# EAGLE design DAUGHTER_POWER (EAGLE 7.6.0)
DAUGHTER CARD POWER

## Sheet 1 of 3: HDK INTERFACE
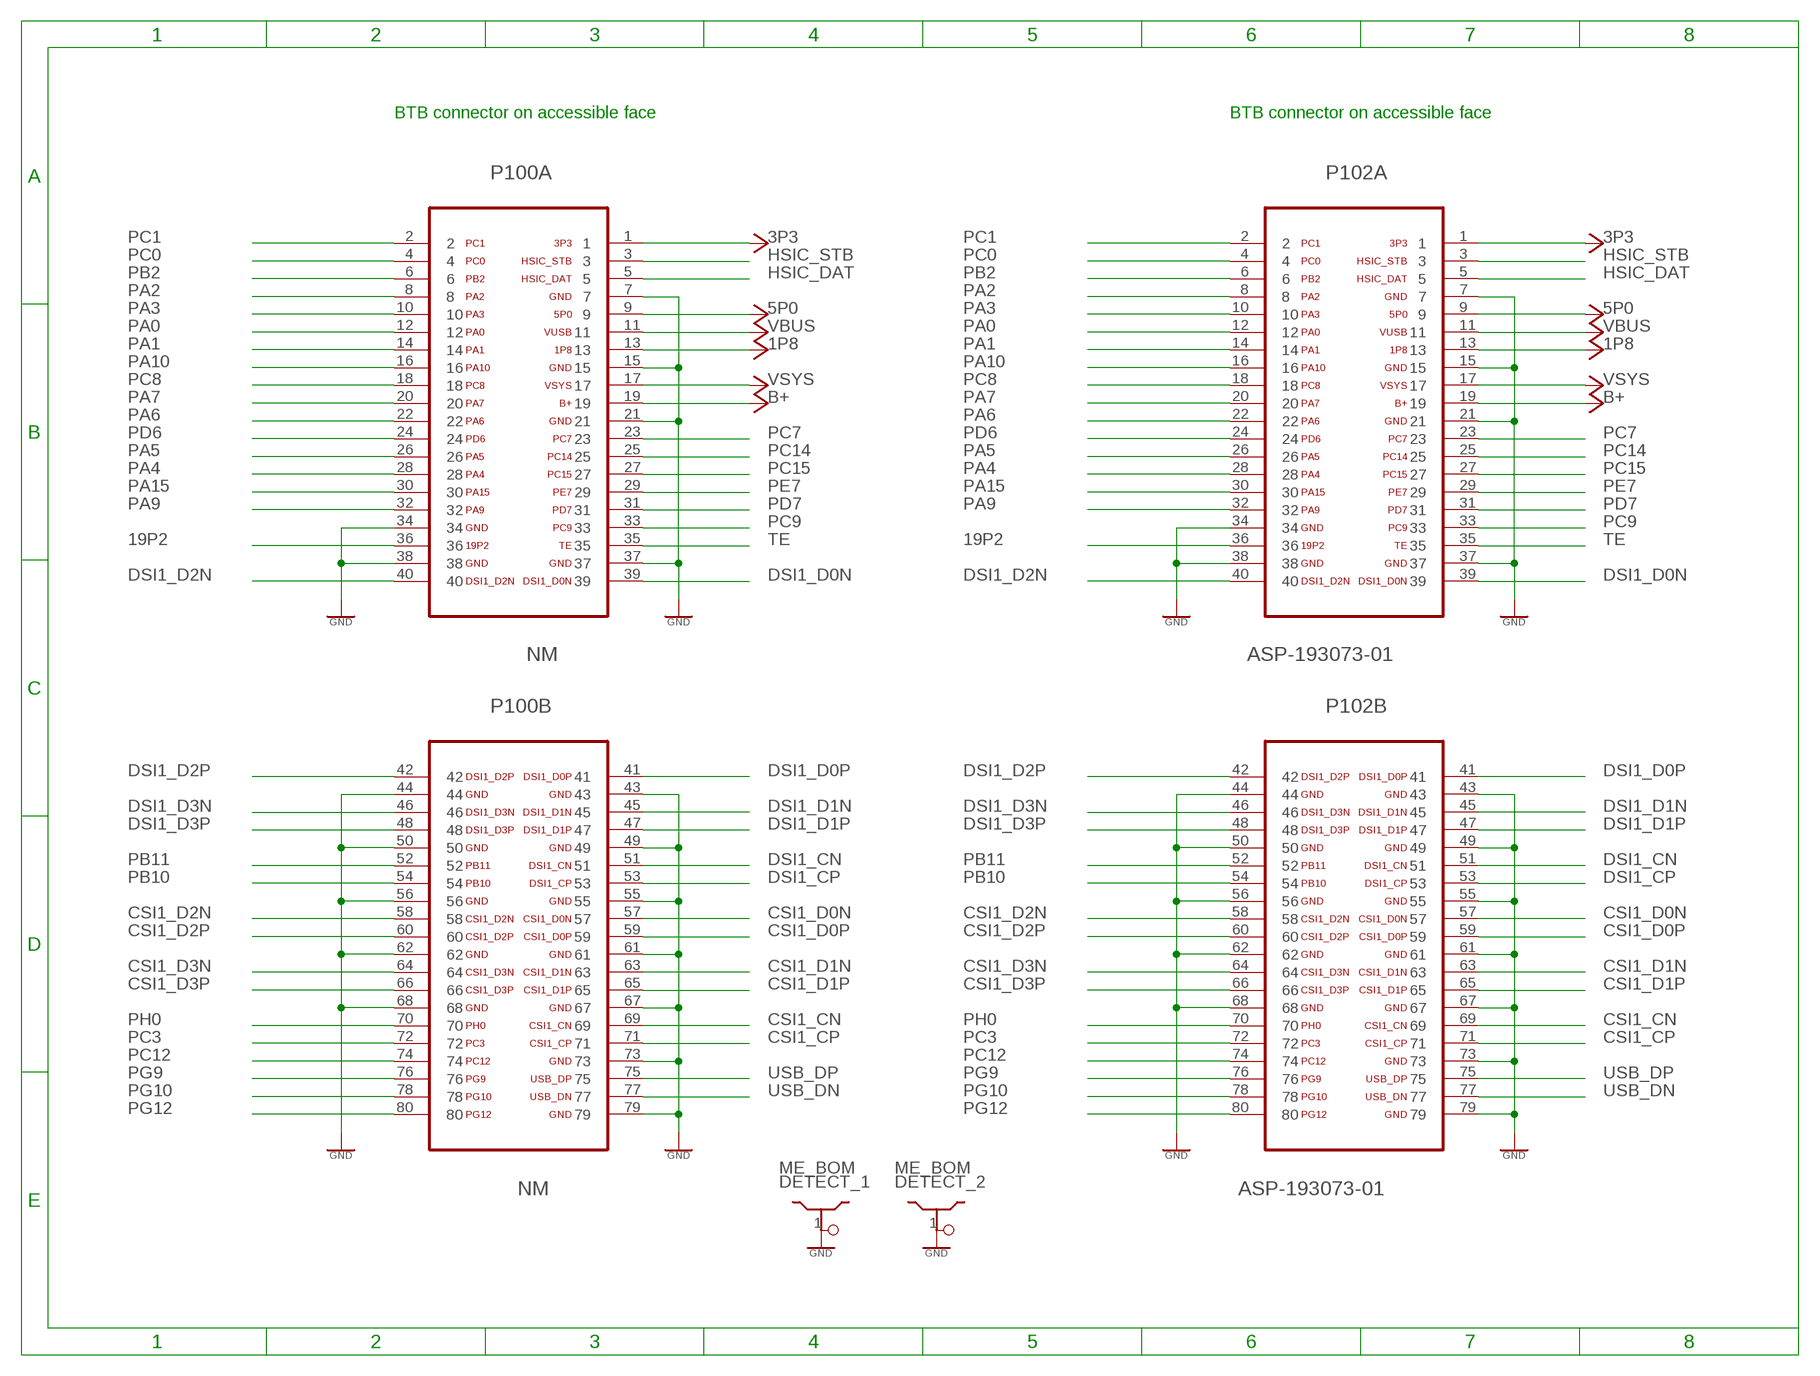
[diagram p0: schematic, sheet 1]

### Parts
DETECT_1  ME_BOM  SHIELDDETECT  [PLUG]
DETECT_2  ME_BOM  SHIELDDETECT  [PLUG]
P100  NM  CLM-140-02-L-D-KGOLD  [CLM-140-02-L-D-K_GOLD]
P102  ASP-193073-01  FTMH-140-02-L-DV-ES-P-TR  [FTMH-140-02-L-DV-ES-P-TR]

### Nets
1P8: P100.13 P102.13 ; also sheet 2,3
3P3: P100.1 P102.1 ; also sheet 2
5P0: P100.9 P102.9
19P2: P100.36 P102.36
B+: P100.19 P102.19
CSI1_CN: P100.69 P102.69
CSI1_CP: P100.71 P102.71
CSI1_D0N: P100.57 P102.57
CSI1_D0P: P100.59 P102.59
CSI1_D1N: P100.63 P102.63
CSI1_D1P: P100.65 P102.65
CSI1_D2N: P100.58 P102.58
CSI1_D2P: P100.60 P102.60
CSI1_D3N: P100.64 P102.64
CSI1_D3P: P100.66 P102.66
DSI1_CN: P100.51 P102.51
DSI1_CP: P100.53 P102.53
DSI1_D0N: P100.39 P102.39
DSI1_D0P: P100.41 P102.41
DSI1_D1N: P100.45 P102.45
DSI1_D1P: P100.47 P102.47
DSI1_D2N: P100.40 P102.40
DSI1_D2P: P100.42 P102.42
DSI1_D3N: P100.46 P102.46
DSI1_D3P: P100.48 P102.48
GND: DETECT_1.1 DETECT_2.1 P100.7 P100.15 P100.21 P100.34 P100.37 P100.38 P100.43 P100.44 P100.49 P100.50 P100.55 P100.56 P100.61 P100.62 P100.67 P100.68 P100.73 P100.79 P102.7 P102.15 P102.21 P102.34 P102.37 P102.38 P102.43 P102.44 P102.49 P102.50 P102.55 P102.56 P102.61 P102.62 P102.67 P102.68 P102.73 P102.79 ; also sheet 2,3
HSIC_DAT: P100.5 P102.5
HSIC_STB: P100.3 P102.3
PA0: P100.12 P102.12
PA1: P100.14 P102.14
PA2: P100.8 P102.8
PA3: P100.10 P102.10
PA4: P100.28 P102.28
PA5: P100.26 P102.26
PA6: P100.22 P102.22
PA7: P100.20 P102.20
PA9: P100.32 P102.32
PA10: P100.16 P102.16
PA15: P100.30 P102.30
PB2: P100.6 P102.6 ; also sheet 3
PB10: P100.54 P102.54 ; also sheet 2,3
PB11: P100.52 P102.52 ; also sheet 2,3
PC0: P100.4 P102.4
PC1: P100.2 P102.2
PC3: P100.72 P102.72
PC7: P100.23 P102.23 ; also sheet 3
PC8: P100.18 P102.18
PC9: P100.33 P102.33
PC12: P100.74 P102.74
PC14: P100.25 P102.25
PC15: P100.27 P102.27
PD6: P100.24 P102.24
PD7: P100.31 P102.31
PE7: P100.29 P102.29
PG9: P100.76 P102.76 ; also sheet 2
PG10: P100.78 P102.78 ; also sheet 3
PG12: P100.80 P102.80 ; also sheet 3
PH0: P100.70 P102.70
TE: P100.35 P102.35
USB_DN: P100.77 P102.77
USB_DP: P100.75 P102.75
VBUS: P100.11 P102.11 ; also sheet 3
VSYS: P100.17 P102.17 ; also sheet 3

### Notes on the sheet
- BTB connector on accessible face | BTB connector on accessible face

## Sheet 2 of 3: Identification
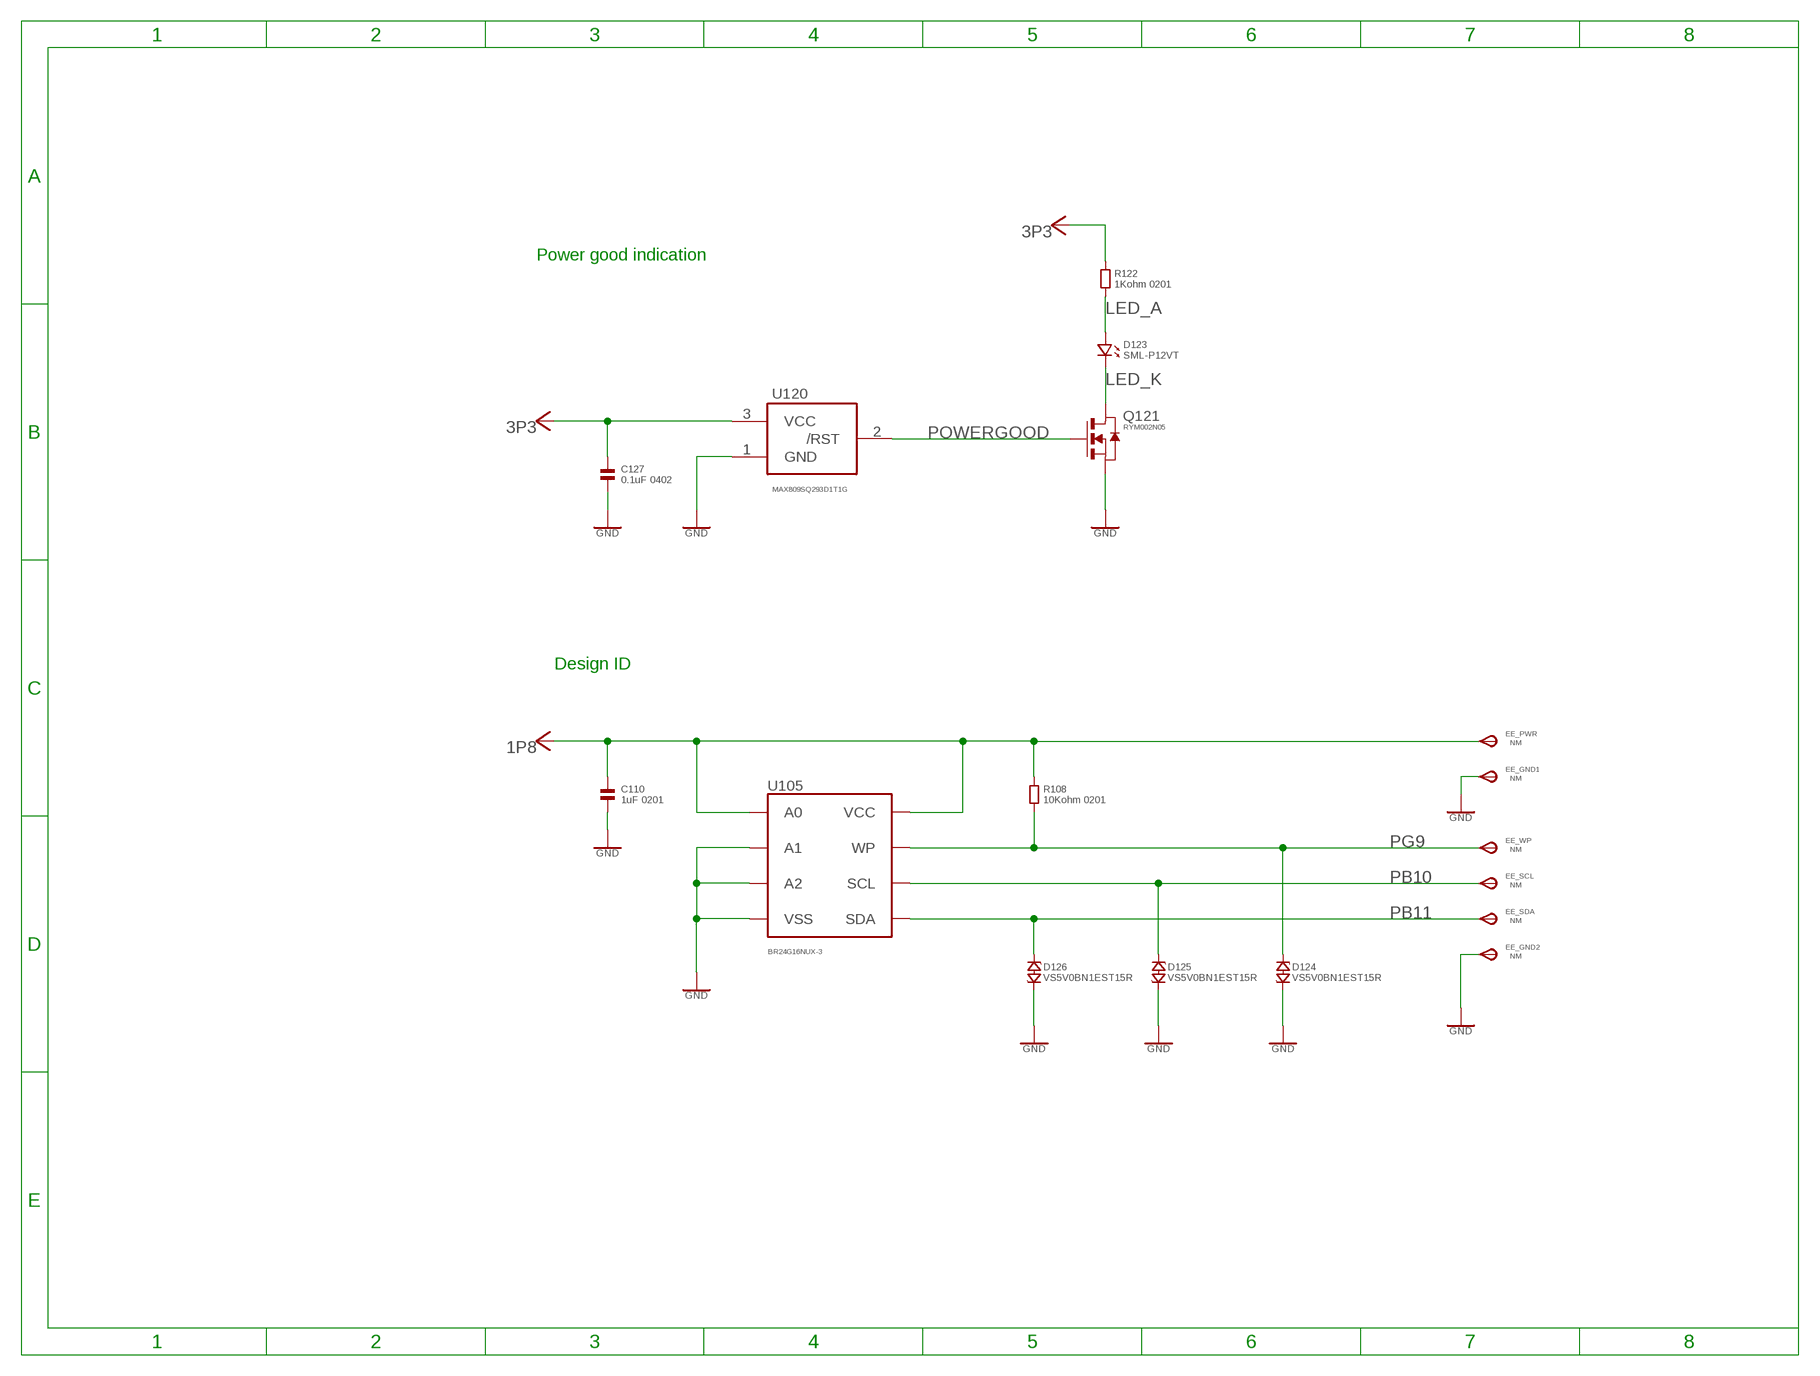
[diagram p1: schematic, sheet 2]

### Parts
C110  1uF 0201  CAPACITOR.0201  [0201]
C127  0.1uF 0402  CAPACITOR.0402  [0402]
D123  SML-P12VT  LED.0503  [0503.LED]
D124  VS5V0BN1EST15R  ESD_VARISTOR.0201  [CHIP_0201]
D125  VS5V0BN1EST15R  ESD_VARISTOR.0201  [CHIP_0201]
D126  VS5V0BN1EST15R  ESD_VARISTOR.0201  [CHIP_0201]
EE_GND1  NM  TPSTP11R  [TP11R]
EE_GND2  NM  TPSTP11R  [TP11R]
EE_PWR  NM  TPSTP11R  [TP11R]
EE_SCL  NM  TPSTP11R  [TP11R]
EE_SDA  NM  TPSTP11R  [TP11R]
EE_WP  NM  TPSTP11R  [TP11R]
Q121  RYM002N05  FET-NRYM002N05  [VMT3]
R108  10Kohm 0201  RESISTOR.0201  [0201]
R122  1Kohm 0201  RESISTOR.0201  [0201]
U105  BR24G16NUX-3  EEPROMDFN8  [DFN-8]
U120  MAX809SQ293D1T1G  MAX809  [SC70-3L]

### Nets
1P8: C110.1 EE_PWR.TP(PP) R108.1 U105.P$1(A0) U105.P$8(VCC) ; also sheet 1,3
3P3: C127.1 R122.1 U120.3(VCC) ; also sheet 1
GND: C110.2 C127.2 D124.P$2 D125.P$2 D126.P$2 EE_GND1.TP(PP) EE_GND2.TP(PP) Q121.2(S) U105.P$2(A1) U105.P$3(A2) U105.P$4(VSS) U105.P$9(VSS) U120.1(GND) ; also sheet 1,3
LED_A: D123.P$1 R122.2
LED_K: D123.P$2 Q121.3(D)
PB10: D125.P$1 EE_SCL.TP(PP) U105.P$6(SCL) ; also sheet 1,3
PB11: D126.P$1 EE_SDA.TP(PP) U105.P$5(SDA) ; also sheet 1,3
PG9: D124.P$1 EE_WP.TP(PP) R108.2 U105.P$7(WP) ; also sheet 1
POWERGOOD: Q121.1(G) U120.2(/RST)

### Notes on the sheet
- Power good indication
- Design ID

## Sheet 3 of 3: BATTERY
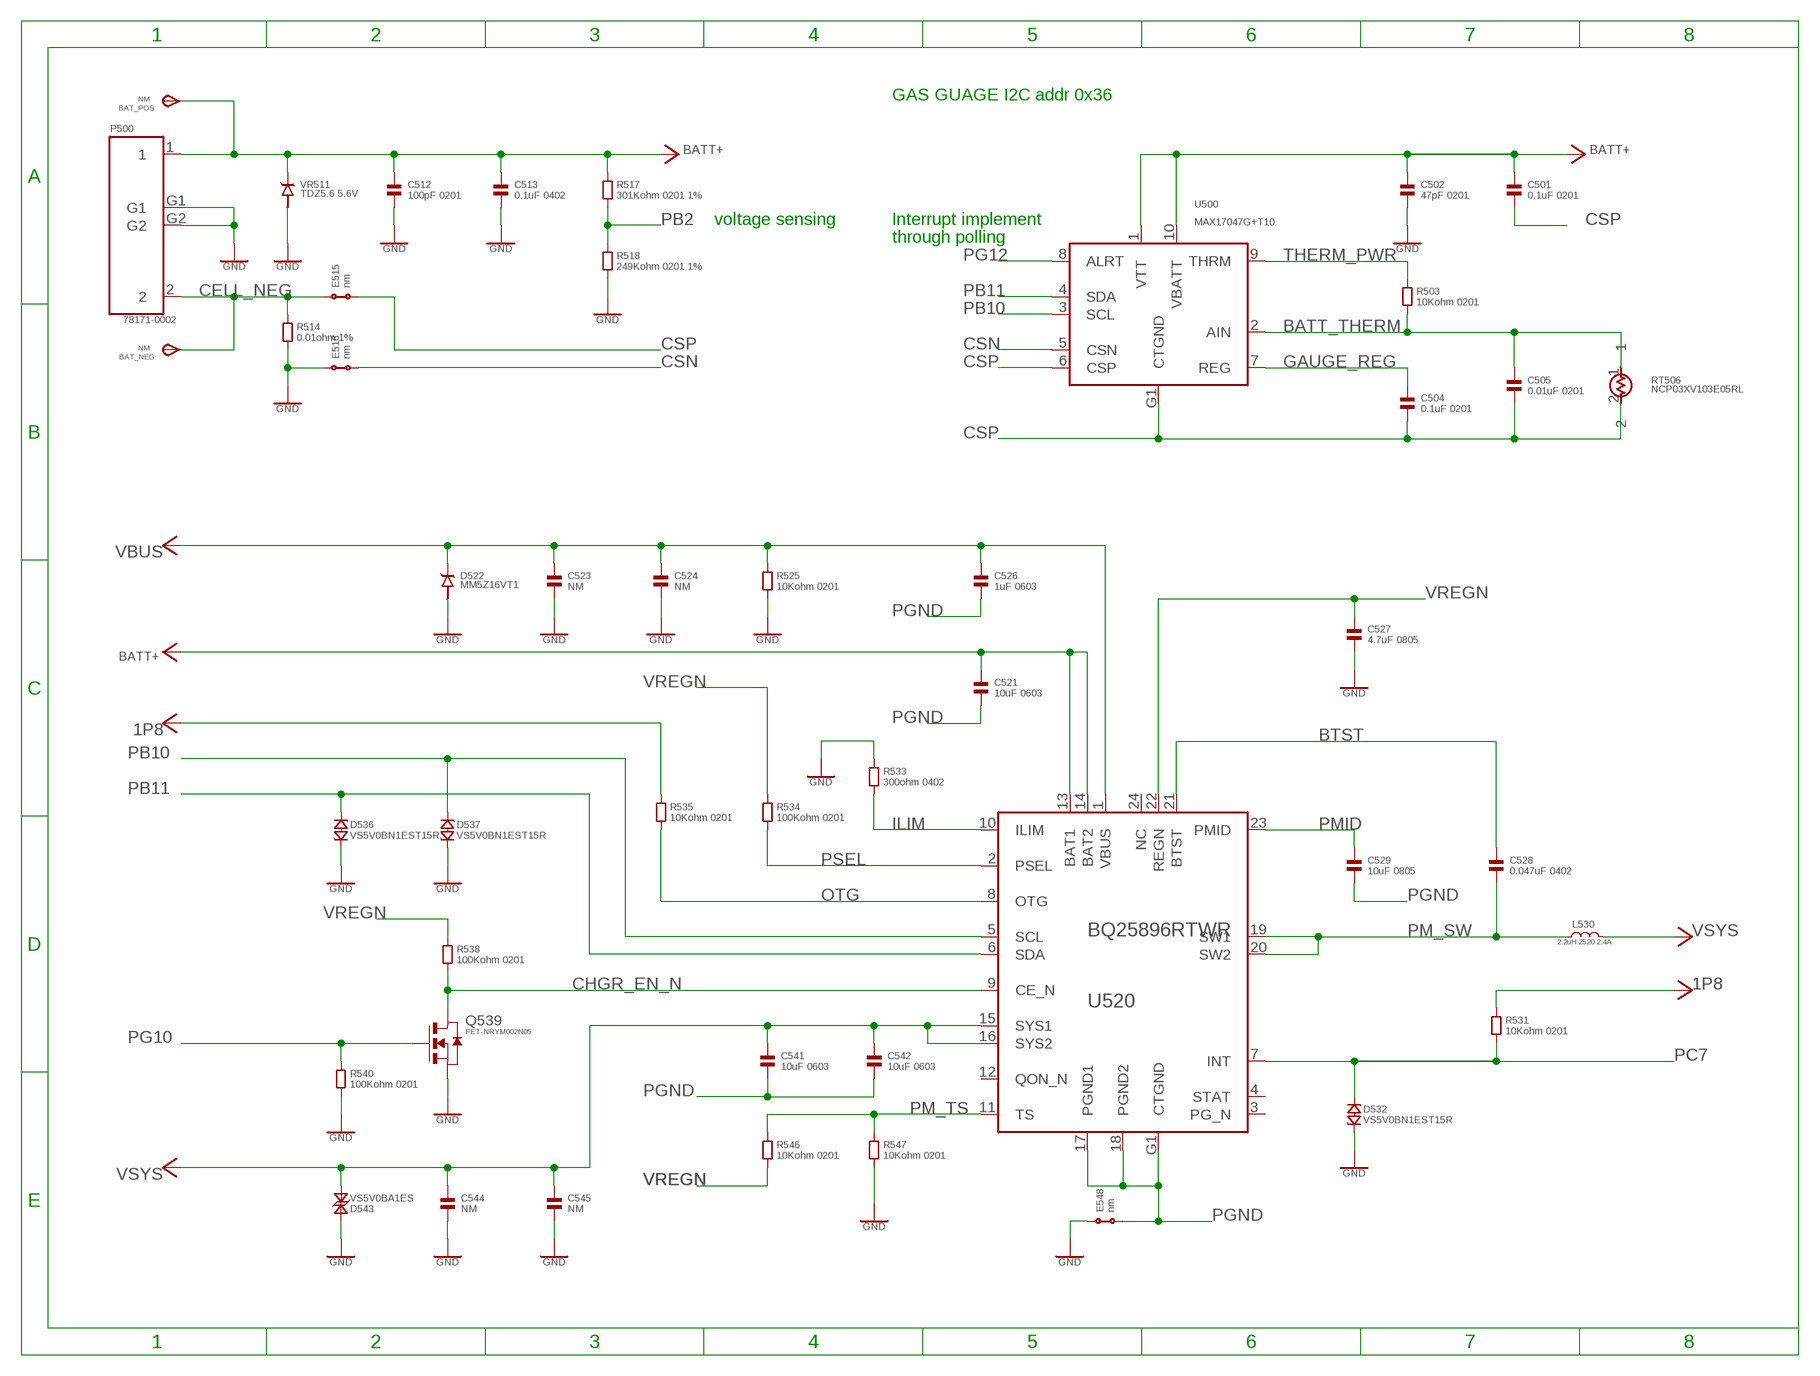
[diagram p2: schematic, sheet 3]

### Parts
BAT_NEG  NM  TPSTP11R  [TP11R]
BAT_POS  NM  TPSTP11R  [TP11R]
C501  0.1uF 0201  CAPACITOR.0201  [0201]
C502  47pF 0201  CAPACITOR.0201  [0201]
C504  0.1uF 0201  CAPACITOR.0201  [0201]
C505  0.01uF 0201  CAPACITOR.0201  [0201]
C512  100pF 0201  CAPACITOR.0201  [0201]
C513  0.1uF 0402  CAPACITOR.0402  [0402]
C521  10uF 0603  CAPACITOR.0603  [0603]
C523  NM  CAPACITOR.0201  [0201]
C524  NM  CAPACITOR.0201  [0201]
C526  1uF 0603  CAPACITOR.0603  [0603]
C527  4.7uF 0805  CAPACITOR.0805  [0805]
C528  0.047uF 0402  CAPACITOR.0402  [0402]
C529  10uF 0805  CAPACITOR.0805  [0805]
C541  10uF 0603  CAPACITOR.0603  [0603]
C542  10uF 0603  CAPACITOR.0603  [0603]
C544  NM  CAPACITOR.0201  [0201]
C545  NM  CAPACITOR.0201  [0201]
D522  MM5Z16VT1  DIODE.SOD523  [SOD523]
D532  VS5V0BN1EST15R  ESD_VARISTOR.0201  [CHIP_0201]
D536  VS5V0BN1EST15R  ESD_VARISTOR.0201  [CHIP_0201]
D537  VS5V0BN1EST15R  ESD_VARISTOR.0201  [CHIP_0201]
D543  VS5V0BA1ES  ESD_TVS.0201  [CHIP_0201]
E515  nm  SHORT_DOT  [SHORT_DOT]
E516  nm  SHORT_DOT  [SHORT_DOT]
E548  nm  SHORT_BAR  [1X4_SHORT]
L530  2.2uH 2520 2.4A  POWER-INDUCTOR  [2520]
P500  78171-0002  CONN_BATT  [CONN_4PIN]
Q539  FET-NRYM002N05  [VMT3]
R503  10Kohm 0201  RESISTOR.0201  [0201]
R514  0.01ohm 1%  RESISTOR.0805  [0805]
R517  301Kohm 0201 1%  RESISTOR.0201  [0201]
R518  249Kohm 0201 1%  RESISTOR.0201  [0201]
R525  10Kohm 0201  RESISTOR.0201  [0201]
R531  10Kohm 0201  RESISTOR.0201  [0201]
R533  300ohm 0402  RESISTOR.0402  [0402]
R534  100Kohm 0201  RESISTOR.0201  [0201]
R535  10Kohm 0201  RESISTOR.0201  [0201]
R538  100Kohm 0201  RESISTOR.0201  [0201]
R540  100Kohm 0201  RESISTOR.0201  [0201]
R546  10Kohm 0201  RESISTOR.0201  [0201]
R547  10Kohm 0201  RESISTOR.0201  [0201]
RT506  NCP03XV103E05RL  THERMISTOR  [0201]
U500  MAX17047G+T10  [DFN3X3_PS0_5P11]
U520  BQ25896RTWR  [QFN4X4PS0_5P25]
VR511  TDZ5.6 5.6V  DIODE  [DIO1_9X1_3]

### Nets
1P8: R531.1 R535.1 ; also sheet 1,2
BATT+: BAT_POS.TP(PP) C501.1 C502.1 C512.1 C513.1 C521.1 P500.1 R517.1 U500.1(VTT) U500.10(VBATT) U520.13(BAT1) U520.14(BAT2) VR511.1
BATT_THERM: C505.1 R503.2 RT506.1 U500.2(AIN)
BTST: C528.1 U520.21(BTST)
CELL_NEG: BAT_NEG.TP(PP) E515.1 P500.2 R514.1
CHGR_EN_N: Q539.3(D) R538.2 U520.9(CE_N)
CSN: E516.2 U500.5(CSN)
CSP: C501.2 C504.2 C505.2 E515.2 RT506.2 U500.6(CSP) U500.G1(CTGND)
GAUGE_REG: C504.1 U500.7(REG)
GND: C502.2 C512.2 C513.2 C523.2 C524.2 C527.2 C544.2 C545.2 D522.2 D532.P$2 D536.P$2 D537.P$2 D543.P$1 E516.1 E548.1 P500.G1 P500.G2 Q539.2(S) R514.2 R518.2 R525.2 R533.1 R540.2 R547.2 VR511.2 ; also sheet 1,2
ILIM: R533.2 U520.10(ILIM)
OTG: R535.2 U520.8(OTG)
PB2: R517.2 R518.1 ; also sheet 1
PB10: D537.P$1 U500.3(SCL) U520.5(SCL) ; also sheet 1,2
PB11: D536.P$1 U500.4(SDA) U520.6(SDA) ; also sheet 1,2
PC7: D532.P$1 R531.2 U520.7(INT) ; also sheet 1
PG10: Q539.1(G) R540.1 ; also sheet 1
PG12: U500.8(ALRT) ; also sheet 1
PGND: C521.2 C526.2 C529.2 C541.2 C542.2 E548.2 U520.17(PGND1) U520.18(PGND2) U520.G1(CTGND)
PM_SW: C528.2 L530.G1 U520.19(SW1) U520.20(SW2)
PM_TS: R546.1 R547.1 U520.11(TS)
PMID: C529.1 U520.23(PMID)
PSEL: R534.2 U520.2(PSEL)
THERM_PWR: R503.1 U500.9(THRM)
VBUS: C523.1 C524.1 C526.1 D522.1 R525.1 U520.1(VBUS) ; also sheet 1
VREGN: C527.1 R534.1 R538.1 R546.2 U520.22(REGN)
VSYS: C541.1 C542.1 C544.1 C545.1 D543.P$2 L530.G2 U520.15(SYS1) U520.16(SYS2) ; also sheet 1
Unconnected: U520.3(PG_N) U520.4(STAT) U520.12(QON_N) U520.24(NC)

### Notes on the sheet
- GAS GUAGE I2C addr 0x36
- voltage sensing | Interrupt implement
- through polling

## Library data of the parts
BAT_NEG BAT_POS EE_GND1 EE_GND2 EE_PWR EE_SCL EE_SDA EE_WP = MOTO_LIB:TPS: TEST Point, 1mm diameter, gold
C110 C127 C501 C502 C504 C505 C512 C513 C521 C523 C524 C526-C529 C541 C542 C544 C545 = MOTO_LIB:CAPACITOR: Ceramic Capacitor, Generic
D123 = MOTO_LIB:LED: LED GENERIC, single, 2 pin; MPN: SML-P12VT; SUPPLIER: ROHM
D124-D126 D532 D536 D537 = MOTO_LIB:ESD_VARISTOR: GENERIC varistor,single, 2 pin; MPN: VS5V0BN1EST15R; SUPPLIER: ROHM
D522 = MOTO_LIB:DIODE: DIODE GENERIC, single, 2 pin; MPN: MM5Z16VT1; SUPPLIER: ON_SEMI
D543 = MOTO_LIB:ESD_TVS: GENERIC TVS,single, 2 pin; MPN: UCLAMP1211Z; SUPPLIER: SEMTECH
DETECT_1 DETECT_2 = MOTO_LIB:SHIELD: Shield, Custom; MPN: refer to ME BOM; SUPPLIER: ref to ME BOM
E515 E516 = MOTO_LIB:SHORT_DOT: short dot, layout feature
E548 = MOTO_LIB:SHORT_BAR: SHORT BAR - layout feature
L530 = MOTO_LIB:POWER-INDUCTOR: Inductor, Power
P100 = MOTO_LIB:CLM-140-02-L-D-K: MICRO SOCKET, 1.0MM pitch, SMD, 2X40WAY, Female; MPN: CLM-140-02-L-D-K; SUPPLIER: SAMTEC
P102 = MOTO_LIB:FTMH-140-02-L-DV-ES-P-TR: MICRO SOCKET, 1.0MM, SMD, 2X40WAY, MALE; MPN: ASP-193073-01; SUPPLIER: SAMTEC
P500 = MOTO_LIB:CONN_BATT: BATTERY connector; MPN: 78171-0002; SUPPLIER: MOLEX
Q121 Q539 = MOTO_LIB:FET-N: Generic NMOS FET; MPN: RYM002N05; SUPPLIER: ROHM
R108 R122 R503 R514 R517 R518 R525 R531 R533-R535 R538 R540 R546 R547 = MOTO_LIB:RESISTOR: Resistor - Generic
RT506 = MOTO_LIB:THERMISTOR: Thmistor, NTC 10Khm 3%, 0201; MPN: NCP03XV103XV103E05RL/NTCG0603UH103HT; SUPPLIER: MURARA/TDK
U105 = MOTO_LIB:EEPROM: I2C EE PROM, 8 pin; MPN: BR24G16NUX-3; SUPPLIER: ROHM
U120 = MOTO_LIB:MAX809: 3-Pin Microprocessor Reset Circuit; MPN: MAX809SQ293D1T1; SUPPLIER: ON-SEMI
U500 = MOTO_LIB:MAX17047G+T10: Fuel Guage; MPN: MAX17047G+T10; SUPPLIER: MAXIM
U520 = MOTO_LIB:BQ25896RTWR: Charging IC, TI BQ2589x; MPN: BQ25896RTWR; SUPPLIER: TI
VR511 = MOTO_LIB:DIODE: DIODE GENERIC, single, 2 pin; MPN: TDZ5.6B; SUPPLIER: ROHM

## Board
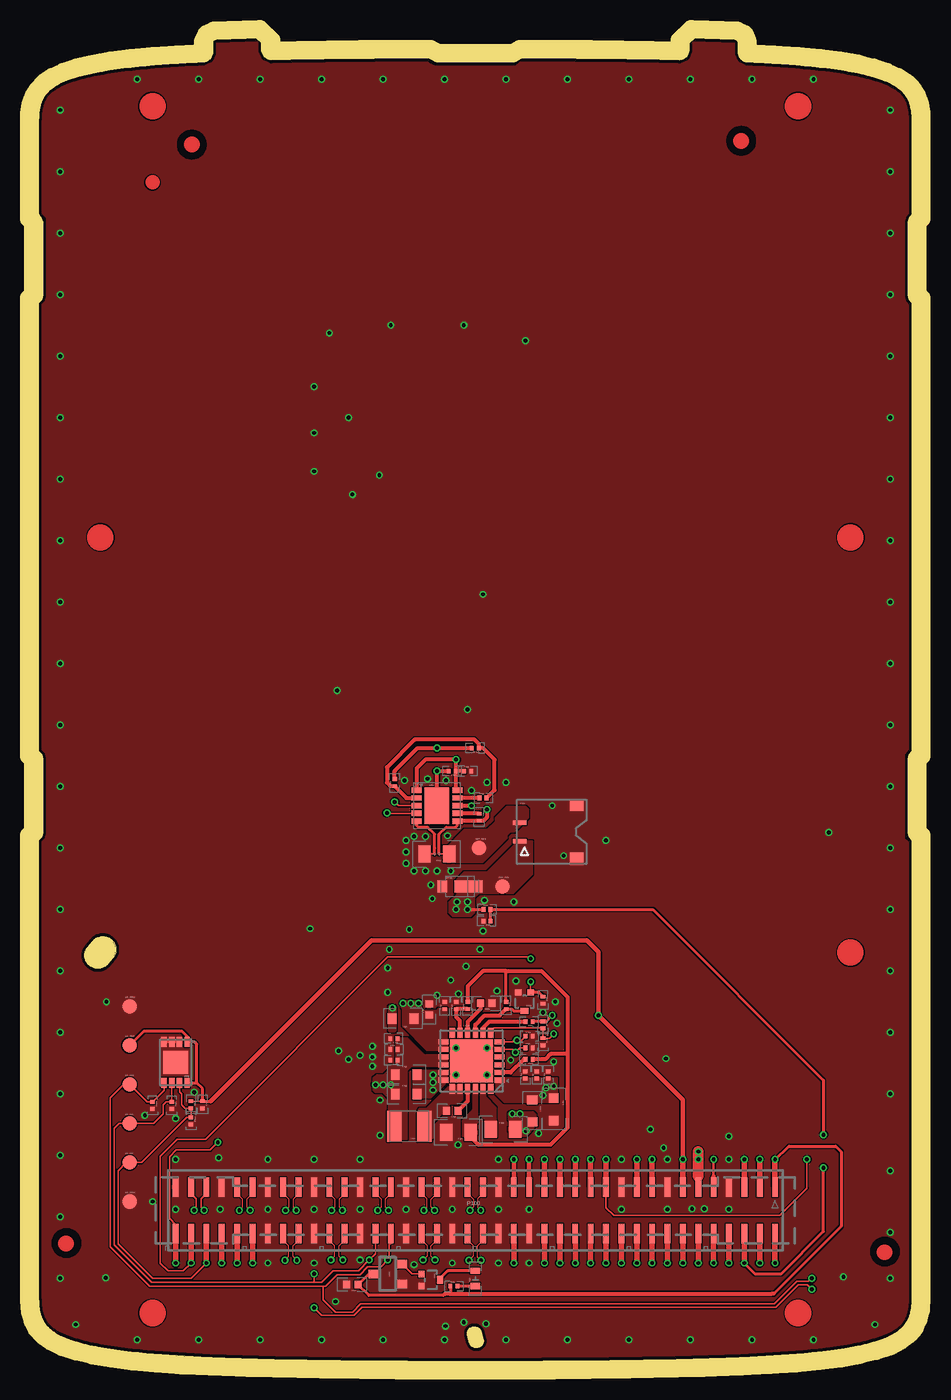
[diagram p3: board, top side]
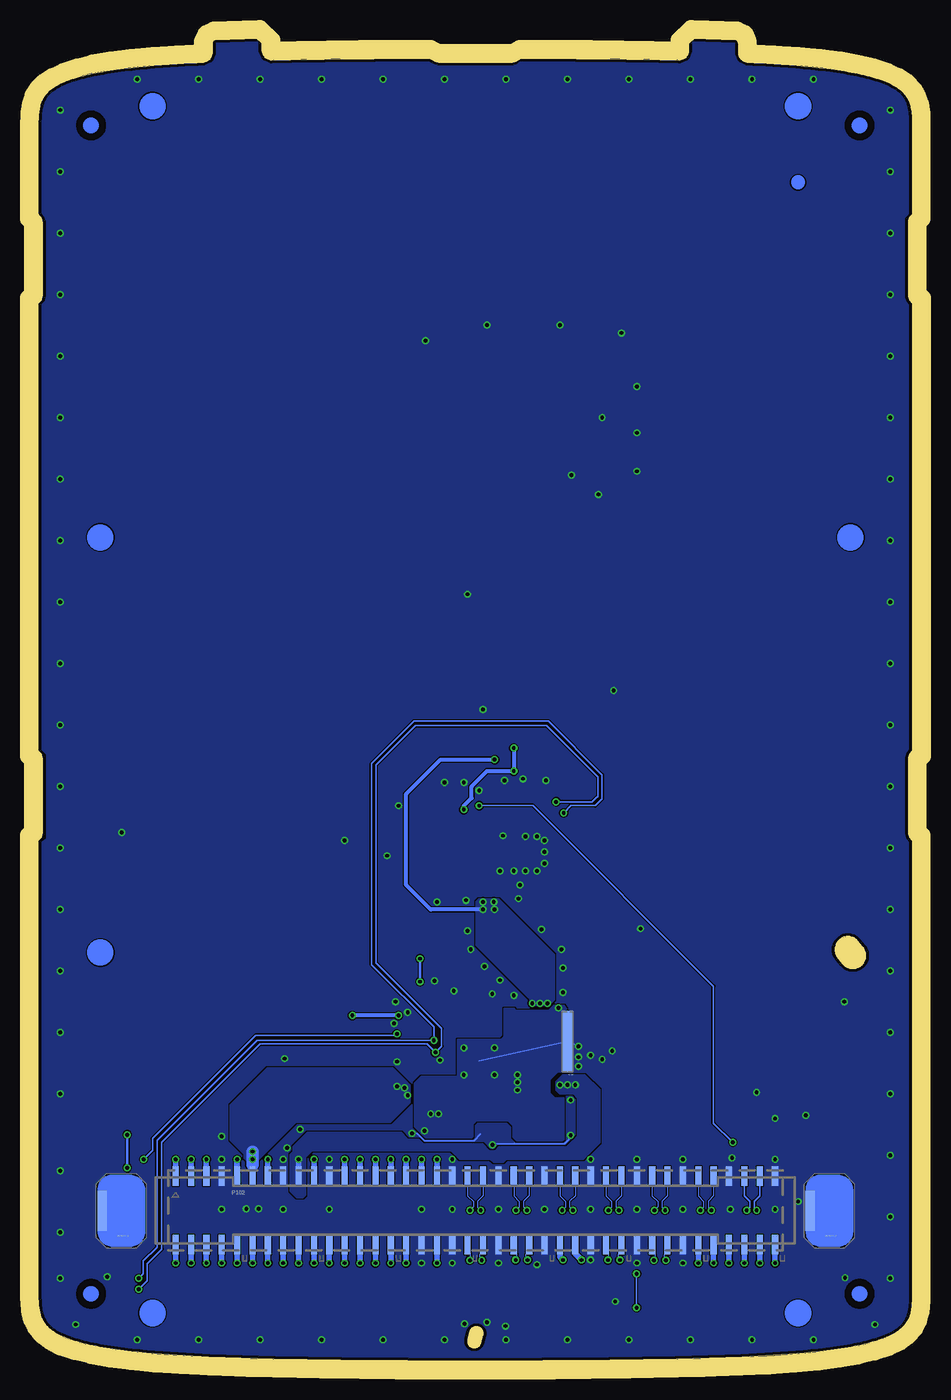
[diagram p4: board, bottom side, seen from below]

Size 56.85 x 86.03 mm. Coordinates in mm from the lower left corner, seen from the top.
Outline: 357 segments
Copper layers (1*16): Top 0.03mm / dielectric 0.787mm / Bottom 0.03mm
Design rules "constraint *": minimum track width 0.08mm, minimum drill 0.25mm, track to track 0.08mm, track to pad 0.08mm, pad to pad 0.08mm, via to via 0.08mm, smd to smd 0.08mm, copper to edge 0.2mm, drill to drill 0.2mm, minimum pad ring 0.1mm, minimum via ring 0.1mm, stop-mask expansion 0mil, vias tented up to drill 0.25mm, thermal gap 0mil
tRestrict: area 54.2,6.2 to 56,7.1; area 54.2,7.1 to 56,8; area 44.8,79.4 to 46.6,80.3; area 44.8,78.5 to 46.6,79.4; area 9.1,79.1 to 10.9,80; area 9.1,78.2 to 10.9,79.1; area 0.9,6.8 to 2.7,7.7; area 0.9,7.7 to 2.7,8.6
bRestrict: area 52.5,4.4 to 54.3,5.3; area 52.5,3.5 to 54.3,4.4; area 2.5,4.4 to 4.3,5.3; area 2.5,3.5 to 4.3,4.4; area 2.5,79.5 to 4.3,80.4; area 2.5,80.4 to 4.3,81.3; area 52.5,80.4 to 54.3,81.3; area 52.5,79.5 to 54.3,80.4
Milling: 125 lines

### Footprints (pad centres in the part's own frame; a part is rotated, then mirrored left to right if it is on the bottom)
TP11R = smd 0.95 x 0.95: TP 0,0
0201 = smd 0.25 x 0.3: 1 -0.23,0; 2 0.23,0
0402 = smd 0.45 x 0.5: 1 -0.37,0; 2 0.37,0
0603 = smd 0.58 x 0.68: 1 -0.71,0; 2 0.71,0
0805 = smd 0.8 x 1.1: 1 -0.8,0; 2 0.8,0
0503.LED = smd 0.4 x 0.6: P$1 -0.495,0; P$2 0.495,0
CHIP_0201 = smd 0.25 x 0.3: P$1 -0.23,0; P$2 0.23,0
SOD523 = smd 0.64 x 0.59: 1 -0.73,0; 2 0.73,0
PLUG = smd 0.6 x 2.6: 1 -1.25,0
SHORT_DOT = smd 0.05 x 0.05: 1 -0.01,0; 2 0.01,0
1X4_SHORT = smd 0.4 x 4: 1 -0.15,0; 2 0.15,0
2520 = smd 0.95 x 2: G1 -0.975,0; G2 0.975,0
CLM-140-02-L-D-K_GOLD = smd 0.38 x 1.27: 1 19.5,1.52; 2 19.5,-1.52; 3 18.5,1.52; 4 18.5,-1.52; 5 17.5,1.52; 6 17.5,-1.52; 7 16.5,1.52; 8 16.5,-1.52; 9 15.5,1.52; 10 15.5,-1.52; 11 14.5,1.52; 12 14.5,-1.52; 13 13.5,1.52; 14 13.5,-1.52; 15 12.5,1.52; 16 12.5,-1.52; 17 11.5,1.52; 18 11.5,-1.52; 19 10.5,1.52; 20 10.5,-1.52; 21 9.5,1.52; 22 9.5,-1.52; 23 8.5,1.52; 24 8.5,-1.52; 25 7.5,1.52; 26 7.5,-1.52; 27 6.5,1.52; 28 6.5,-1.52; 29 5.5,1.52; 30 5.5,-1.52; 31 4.5,1.52; 32 4.5,-1.52; 33 3.5,1.52; 34 3.5,-1.52; 35 2.5,1.52; 36 2.5,-1.52; 37 1.5,1.52; 38 1.5,-1.52; 39 0.5,1.52; 40 0.5,-1.52; 41 -0.5,1.52; 42 -0.5,-1.52; 43 -1.5,1.52; 44 -1.5,-1.52; 45 -2.5,1.52; 46 -2.5,-1.52; 47 -3.5,1.52; 48 -3.5,-1.52; 49 -4.5,1.52; 50 -4.5,-1.52; 51 -5.5,1.52; 52 -5.5,-1.52; 53 -6.5,1.52; 54 -6.5,-1.52; 55 -7.5,1.52; 56 -7.5,-1.52; 57 -8.5,1.52; 58 -8.5,-1.52; 59 -9.5,1.52; 60 -9.5,-1.52; 61 -10.5,1.52; 62 -10.5,-1.52; 63 -11.5,1.52; 64 -11.5,-1.52; 65 -12.5,1.52; 66 -12.5,-1.52; 67 -13.5,1.52; 68 -13.5,-1.52; 69 -14.5,1.52; 70 -14.5,-1.52; 71 -15.5,1.52; 72 -15.5,-1.52; 73 -16.5,1.52; 74 -16.5,-1.52; 75 -17.5,1.52; 76 -17.5,-1.52; 77 -18.5,1.52; 78 -18.5,-1.52; 79 -19.5,1.52; 80 -19.5,-1.52
FTMH-140-02-L-DV-ES-P-TR = smd 0.4 x 1.263: 1 -19.5,2.223; 2 -19.5,-2.223; 3 -18.5,2.223; 4 -18.5,-2.223; 5 -17.5,2.223; 6 -17.5,-2.223; 7 -16.5,2.223; 8 -16.5,-2.223; 9 -15.5,2.223; 10 -15.5,-2.223; 11 -14.5,2.223; 12 -14.5,-2.223; 13 -13.5,2.223; 14 -13.5,-2.223; 15 -12.5,2.223; 16 -12.5,-2.223; 17 -11.5,2.223; 18 -11.5,-2.223; 19 -10.5,2.223; 20 -10.5,-2.223; 21 -9.5,2.223; 22 -9.5,-2.223; 23 -8.5,2.223; 24 -8.5,-2.223; 25 -7.5,2.223; 26 -7.5,-2.223; 27 -6.5,2.223; 28 -6.5,-2.223; 29 -5.5,2.223; 30 -5.5,-2.223; 31 -4.5,2.223; 32 -4.5,-2.223; 33 -3.5,2.223; 34 -3.5,-2.223; 35 -2.5,2.223; 36 -2.5,-2.223; 37 -1.5,2.223; 38 -1.5,-2.223; 39 -0.5,2.223; 40 -0.5,-2.223; 41 0.5,2.223; 42 0.5,-2.223; 43 1.5,2.223; 44 1.5,-2.223; 45 2.5,2.223; 46 2.5,-2.223; 47 3.5,2.223; 48 3.5,-2.223; 49 4.5,2.223; 50 4.5,-2.223; 51 5.5,2.223; 52 5.5,-2.223; 53 6.5,2.223; 54 6.5,-2.223; 55 7.5,2.223; 56 7.5,-2.223; 57 8.5,2.223; 58 8.5,-2.223; 59 9.5,2.223; 60 9.5,-2.223; 61 10.5,2.223; 62 10.5,-2.223; 63 11.5,2.223; 64 11.5,-2.223; 65 12.5,2.223; 66 12.5,-2.223; 67 13.5,2.223; 68 13.5,-2.223; 69 14.5,2.223; 70 14.5,-2.223; 71 15.5,2.223; 72 15.5,-2.223; 73 16.5,2.223; 74 16.5,-2.223; 75 17.5,2.223; 76 17.5,-2.223; 77 18.5,2.223; 78 18.5,-2.223; 79 19.5,2.223; 80 19.5,-2.223
CONN_4PIN = smd 0.88 x 0.3: 1 -2.075,-0.6; 2 -2.075,0.6 | smd 0.9 x 0.8: G1 1.645,-1.75; G2 1.645,1.75
VMT3 = smd 0.42 x 0.4: 1 -0.4,-0.6; 2 0.4,-0.6 | smd 0.52 x 0.4: 3 0,0.6
DFN-8 = smd 0.35 x 0.65: P$1 -0.75,-1.325; P$2 -0.25,-1.325; P$3 0.25,-1.325; P$4 0.75,-1.325; P$5 0.75,1.325; P$6 0.25,1.325; P$7 -0.25,1.325; P$8 -0.75,1.325 | smd 1.6 x 1.5: P$9 0,0
SC70-3L = smd 0.55 x 0.63: 1 -0.65,-0.94; 3 0,0.94 | smd 0.555 x 0.63: 2 0.65,-0.94
DFN3X3_PS0_5P11 = smd 0.65 x 0.35: 1 -1.325,1; 2 -1.325,0.5; 3 -1.325,0; 4 -1.325,-0.5; 5 -1.325,-1; 6 1.325,-1; 7 1.325,-0.5; 8 1.325,0; 9 1.325,0.5; 10 1.325,1 | smd 1.6 x 2.4: G1 0,0
QFN4X4PS0_5P25 = smd 0.65 x 0.33: 1 1.825,-1.25; 2 1.825,-0.75; 3 1.825,-0.25; 4 1.825,0.25; 5 1.825,0.75; 6 1.825,1.25; 13 -1.825,1.25; 14 -1.825,0.75; 15 -1.825,0.25; 16 -1.825,-0.25; 17 -1.825,-0.75; 18 -1.825,-1.25 | smd 0.33 x 0.65: 7 1.25,1.825; 8 0.75,1.825; 9 0.25,1.825; 10 -0.25,1.825; 11 -0.75,1.825; 12 -1.25,1.825; 19 -1.25,-1.825; 20 -0.75,-1.825; 21 -0.25,-1.825; 22 0.25,-1.825; 23 0.75,-1.825; 24 1.25,-1.825 | smd 2.8 x 2.8: G1 0,0
DIO1_9X1_3 = smd 1.8 x 0.8: 1 0.55,0 | smd 0.6 x 0.8: 2 -1.15,0

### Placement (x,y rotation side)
BAT_NEG  28.67,33.37 0 top
BAT_POS  30.17,30.87 0 top
C110  10.67,16.67 270 top
C127  20.42,4.97 180 top
C501  26.92,38.37 180 top
C502  27.92,38.37 0 top
C504  28.67,35.37 270 top
C505  23.17,37.62 90 top
C512  26.42,23.12 90 top
C513  25.42,22.87 90 top
C521  23.72,22.27 180 top
C523  32.42,18.62 90 top
C524  31.67,18.62 90 top
C526  32.12,16.27 270 top
C527  27.32,14.87 180 top
C528  26.92,16.27 180 top
C529  30.22,15.07 0 top
C541  23.92,18.62 0 top
C542  23.92,17.37 0 top
C544  23.12,19.57 180 top
C545  23.12,20.97 180 top
D123  28.42,5.37 90 top
D124  9.92,15.62 270 top
D125  8.67,16.62 270 top
D126  7.42,16.62 270 top
D522  33.52,16.37 270 top
D532  32.82,20.77 270 top
D536  31.92,21.12 0 top
D537  31.92,20.37 0 top
D543  23.12,20.27 0 top
DETECT_1  51.45,9.77 0 bottom
DETECT_2  5.39,9.77 0 bottom
E515  26.07,32.97 0 top
E516  25.77,32.97 0 top
E548  22.42,20.77 180 bottom
EE_GND1  5.92,10.37 0 top
EE_GND2  5.92,23.07 0 top
EE_PWR  5.92,20.53 0 top
EE_SCL  5.92,15.45 0 top
EE_SDA  5.92,17.99 0 top
EE_WP  5.92,12.91 0 top
L530  24.12,15.27 180 top
P100  28.42,9.8 0 top
P102  28.42,9.8 0 bottom
P500  33.37,34.42 0 top
Q121  25.52,5.27 270 top
Q539  31.62,23.37 180 top
R108  9.92,16.67 270 top
R122  27.02,4.87 0 top
R503  28.92,36.62 0 top
R514  25.92,32.97 180 top
R517  29.17,29.37 0 top
R518  29.17,28.62 180 top
R525  33.17,18.62 90 top
R531  32.82,21.87 270 top
R533  29.12,23.27 180 top
R534  31.92,19.62 180 top
R535  31.92,22.07 180 top
R538  30.42,23.12 270 top
R540  32.82,23.47 270 top
R546  27.92,23.12 90 top
R547  27.17,23.12 90 top
RT506  28.42,39.87 180 top
U105  8.92,19.42 180 top
U120  22.72,5.67 90 top
U500  25.92,36.12 0 top
U520  28.17,19.52 0 top
VR511  27.42,30.87 0 top

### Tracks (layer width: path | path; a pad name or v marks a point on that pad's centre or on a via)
1P8  (via drill 0.25)
  Top 0.1: R108.1 C110.1
  Top 0.2: EE_PWR.TP 6.86,21.47 9.32,21.47 9.67,21.12 U105.P$1 10.15,20.75 10.3,20.6 10.3,18.1 | U105.P$8 10.3,18.1 | 10.3,18.1 10.67,17.72 C110.1 11.2,16.9 | R535.1 32.18,22.1 R531.1 33.05,22.1 v33.42,22.47
  Top 0.3: 11.2,16.9 21.67,27.37 35.67,27.37 36.42,26.62 v36.42,22.47 41.92,16.97 v41.92,13.12
  Top 0.35: P100.13 v41.92,13.12
  Bottom 0.25: v33.42,22.47 v36.42,22.47
  Bottom 0.35: P102.13 v41.92,13.12
3P3  (via drill 0.25)
  Top 0.2: U120.3 21.49,5.67 C127.1 21.49,4.27 26.32,4.27 26.42,4.37 | R122.1 26.79,4.37 | 47.92,13.07 48.82,13.97 51.87,13.97 52.22,13.62 52.22,8.77 47.83,4.38
  Top 0.25: 26.42,4.37 26.79,4.37 47.67,4.37 47.83,4.38
  Top 0.35: P100.1 v47.92,13.12 47.92,13.07
  Bottom 0.35: P102.1 v47.92,13.12
5P0  (via drill 0.25)
  Top 0.15: v43.92,13.12 P102.9
  Top 0.25: P100.9 P102.9
  Bottom 0.4: P102.9 v43.92,13.12
19P2  (via drill 0.25)
  Top 0.35: P100.36 v30.92,6.37
  Bottom 0.35: v30.92,6.37 P102.36
B+  (via drill 0.25)
  Top 0.35: P100.19 v38.92,13.12
  Bottom 0.35: v38.92,13.12 P102.19
BATT+  (via drill 0.25)
  Top 0.1: v27.17,39.12 27.15,39.1
  Top 0.2: v27.92,29.37 R517.1
  Top 0.25: U500.1 24.6,38.55 25.17,39.12 v27.17,39.12 | C501.1 27.15,39.1 | C501.1 27.15,37.22 U500.10 | C502.1 C501.1
  Bottom 0.25: v27.92,29.37 31.32,29.37 32.92,30.97 32.92,36.87 30.67,39.12 v27.17,39.12
  other vias: 27.92,29.87 27.22,29.87 27.17,29.37 23.72,23.27 24.22,23.27 24.72,23.27
  pour Bottom: 23.27,23.52 23.67,23.12 24.82,23.12 24.87,23.17 24.87,23.62 24.92,23.62 28.37,27.07 28.37,29.87 28.17,30.07 26.92,30.07 23.27,26.42
  pour Top: 32.12,33.82 30.97,33.82 30.97,33.57 29.22,31.82 27.72,31.82 27.22,31.32 27.22,30.32 26.72,29.82 26.72,29.17 26.97,28.92 28.12,28.92 28.37,29.17 28.37,30.17 28.62,30.42 30.87,30.42 32.12,31.67
  pour Top: 23.67,23.42 24.77,23.42 24.87,23.32 24.87,22.92 24.97,22.82 25.92,22.82 26.02,22.92 26.57,22.92 26.57,20.22 25.27,20.22 23.67,21.82 23.67,22.92 23.62,22.97 23.62,23.37
BATT_THERM
  Top 0.25: R503.2 29.67,37.14 29.67,39.12 28.92,39.87 RT506.1 28.65,40.14 28.37,40.42 24.47,40.42 22.67,38.62 22.67,37.62 22.9,37.39 C505.1 23.94,36.62 U500.2
BTST
  Top 0.25: U520.21 27.92,16.9 C528.1
CELL_NEG
  Top 0.1: E515.1 R514.1 E515.1
  pour Top: 27.72,34.57 29.22,34.57 29.72,35.07 29.72,35.32 30.47,36.07 31.67,36.07 31.87,35.87 31.87,35.37 30.92,34.42 30.67,34.42 30.47,34.22 30.47,34.02 28.87,32.42 26.47,32.42 26.47,33.32
CHGR_EN_N
  Top 0.2: R538.2 30.8,22.89 30.92,22.77 Q539.3
  Top 0.25: U520.9 28.42,21.87 29.02,22.47 30,22.47 R538.2
CSI1_CN  (via drill 0.25)
  Top 0.08: P100.69 13.92,10.9 13.57,10.55 13.57,10 v13.77,9.8
  Bottom 0.08: P102.69 13.92,10.75 13.57,10.4 13.57,10 v13.77,9.8
CSI1_CP  (via drill 0.25)
  Top 0.08: P100.71 12.92,10.9 13.29,10.53 13.29,10.02 v13.07,9.8
  Bottom 0.08: P102.71 12.92,10.75 13.27,10.4 13.27,10 v13.07,9.8
CSI1_D0N  (via drill 0.25)
  Top 0.08: P100.57 19.92,10.9 19.55,10.53 19.55,10.02 v19.77,9.8
  Bottom 0.08: P102.57 19.92,10.75 19.57,10.4 19.57,10 v19.77,9.8
CSI1_D0P  (via drill 0.25)
  Top 0.08: P100.59 18.92,10.9 19.27,10.55 19.27,10 v19.07,9.8
  Bottom 0.08: P102.59 18.92,10.75 19.29,10.38 19.29,10.02 v19.07,9.8
CSI1_D1N  (via drill 0.25)
  Top 0.08: P100.63 16.92,10.9 16.55,10.53 16.55,10.02 v16.77,9.8
  Bottom 0.08: P102.63 16.92,10.75 16.55,10.38 16.55,10.02 v16.77,9.8
CSI1_D1P  (via drill 0.25)
  Top 0.08: 15.92,10.9 16.27,10.55 16.27,10 v16.07,9.8
  Top 0.1: P100.65 15.92,10.9
  Bottom 0.08: P102.65 15.92,10.75 16.27,10.4 16.27,10 v16.07,9.8
CSI1_D2N  (via drill 0.25)
  Top 0.08: P100.58 19.92,7.85 19.57,7.5 19.57,6.8 v19.8,6.58
  Bottom 0.08: P102.58 19.92,7.17 19.72,6.97 19.72,6.65 v19.8,6.58
CSI1_D2P  (via drill 0.25)
  Top 0.08: P100.60 18.92,7.85 19.27,7.5 19.27,6.82 v19.03,6.58
  Bottom 0.08: P102.60 18.92,7.15 19.12,6.95 19.12,6.67 v19.03,6.58
CSI1_D3N  (via drill 0.25)
  Top 0.08: P100.64 16.92,7.85 16.57,7.5 16.57,6.8 v16.81,6.57
  Bottom 0.08: P102.64 16.92,7.12 16.72,6.92 16.72,6.65 v16.81,6.57
CSI1_D3P  (via drill 0.25)
  Top 0.08: P100.66 15.92,7.85 16.27,7.5 16.27,6.8 v16.03,6.57
  Bottom 0.08: P102.66 15.92,7.12 16.12,6.92 16.12,6.65 v16.03,6.57
CSN
  Top 0.1: E516.2 25.77,33.37
  Top 0.2: E516.2 25.77,33.37 25.77,34.27 25.32,34.72 24.72,34.72 24.6,34.85 U500.5
CSP  (via drill 0.25)
  Top 0.1: 27.27,35.14 U500.6 | E515.2
  Top 0.2: E515.2 26.07,34.27 26.52,34.72 27.12,34.72 27.25,34.85 U500.6
  Top 0.25: 27.27,35.14 C504.2 28.94,35.14 29.17,35.37 v29.17,35.87 | C501.2 v25.92,38.37 U500.G1 | RT506.2 v25.92,39.87 24.67,39.87 23.17,38.37 C505.2
  Bottom 0.25: v29.17,35.87 29.17,36.12 28.67,36.62 28.67,37.37 27.67,38.37 v25.92,38.37 v25.92,39.87
DSI1_CN  (via drill 0.25)
  Top 0.08: 22.92,10.9 22.55,10.53 22.55,10.02 v22.77,9.8
  Top 0.1: P100.51 22.92,10.9
  Bottom 0.08: P102.51 22.92,10.75 22.57,10.4 22.57,10 v22.77,9.8
DSI1_CP  (via drill 0.25)
  Top 0.08: P100.53 21.92,10.9 22.27,10.55 22.27,10 v22.07,9.8
  Bottom 0.08: P102.53 21.92,10.75 22.29,10.39 22.29,10.02 v22.07,9.8
DSI1_D0N  (via drill 0.25)
  Top 0.08: P100.39 28.92,10.9 28.57,10.55 28.57,10 v28.77,9.8
  Bottom 0.08: P102.39 28.92,10.75 28.55,10.38 28.55,10.02 v28.77,9.8
DSI1_D0P  (via drill 0.25)
  Top 0.08: P100.41 27.92,10.9 28.29,10.53 28.29,10.02 v28.07,9.8
  Bottom 0.08: P102.41 27.92,10.75 28.27,10.4 28.27,10 v28.07,9.8
DSI1_D1N  (via drill 0.25)
  Top 0.08: P100.45 25.92,10.9 25.55,10.53 25.55,10.02 v25.77,9.8
  Bottom 0.08: P102.45 25.92,10.75 25.57,10.4 25.57,10 v25.77,9.8
DSI1_D1P  (via drill 0.25)
  Top 0.08: P100.47 24.92,10.9 25.27,10.55 25.27,10 v25.07,9.8
  Bottom 0.08: P102.47 24.92,10.75 25.29,10.38 25.29,10.02 v25.07,9.8
DSI1_D2N  (via drill 0.25)
  Top 0.08: P100.40 28.92,7.85 28.57,7.5 28.57,6.76 v28.78,6.56
  Bottom 0.08: P102.40 28.92,7.17 28.72,6.97 28.72,6.61 v28.78,6.56
DSI1_D2P  (via drill 0.25)
  Top 0.08: P100.42 27.92,7.85 28.29,7.48 28.29,6.84 v28.01,6.56
  Bottom 0.08: P102.42 27.92,7.15 28.12,6.95 28.12,6.67 v28.01,6.56
DSI1_D3N  (via drill 0.25)
  Top 0.08: P100.46 25.92,7.87 25.56,7.5 25.55,6.82 v25.8,6.58
  Bottom 0.08: P102.46 25.92,7.17 25.72,6.97 25.72,6.65 v25.8,6.58
DSI1_D3P  (via drill 0.25)
  Top 0.08: P100.48 24.92,7.87 25.27,7.52 25.27,6.82 v25.03,6.58
  Bottom 0.08: P102.48 24.92,7.15 25.12,6.95 25.12,6.67 v25.03,6.58
GAUGE_REG
  Top 0.1: U500.7 27.42,35.6
  Top 0.25: C504.1 27.42,35.6 27.27,35.6
GND  (via drill 0.25)
  Top 0.1: E516.1 25.72,32.97 | 25.72,32.97 25.17,32.97 | 25.17,32.97 R514.2 | 25.72,32.97 E516.1 25.17,32.97
  Top 0.2: U105.P$4 U105.P$3 U105.P$2
  Bottom 0.1: v32.54,14.81 32.21,14.81 31.72,14.32 28.52,14.32 28.07,14.77 | v27.3,14.07 27.25,14.12 25.87,14.12 | 25.92,14.17 25.87,14.12 | 25.87,14.12 22.62,14.12 22.32,14.42 | E548.1 v21.72,20.47
  other vias: 14.42,1.37 10.42,1.37 6.42,1.37 22.42,1.37 18.42,1.37 26.42,1.37 30.42,1.37 34.42,1.37 38.42,1.37 42.42,1.37 46.42,1.37 50.42,1.37 54.42,2.37 55.42,8.37 55.42,5.37 55.42,12.37 55.42,17.37 55.42,21.37 55.42,25.37 55.42,29.37 55.42,33.37 55.42,37.37 55.42,41.37 55.42,45.37 55.42,49.37 55.42,53.37 55.42,57.37 55.42,61.37 55.42,65.37 55.42,69.37 55.42,73.37 55.42,77.37 55.42,81.37 50.42,83.37 46.42,83.37 42.42,83.37 38.42,83.37 34.42,83.37 30.42,83.37 26.42,83.37 22.42,83.37 18.42,83.37 14.42,83.37 10.42,83.37 6.42,83.37 1.42,81.37 1.42,77.37 1.42,73.37 1.42,69.37 1.42,65.37 1.42,61.37 1.42,57.37 1.42,53.37 1.42,49.37 1.42,45.37 1.42,41.37 1.42,37.37 1.42,33.37 1.42,29.37 1.42,25.37 4.42,23.37 1.42,21.37 1.42,17.37 1.42,13.37 1.42,9.37 1.42,5.37 2.42,2.37 8.92,13.12 11.72,13.22 14.92,13.12 17.92,13.12 20.92,13.12 29.92,13.12 29.92,9.87 31.92,9.87 26.92,9.87 23.92,9.87 20.92,9.87 17.92,9.87 14.92,9.87 11.82,9.87 8.92,9.87 7.42,10.37 8.92,15.77 10.12,17.47 14.92,6.37 17.92,6.37 20.92,6.57 24.42,6.27 26.92,6.37 29.92,6.37 31.92,6.37 44.92,9.87 42.52,9.9 43.32,9.9 40.92,9.87 37.92,9.87 37.92,13.12 40.92,13.12 44.92,13.12 6.92,15.97 29.12,2.42 27.67,2.52 26.47,2.27 52.37,5.47 4.37,5.42 31.67,66.37 27.67,67.37 22.92,67.37 18.92,66.87 17.92,63.37 17.92,60.37 20.17,61.37 17.92,57.87 20.42,56.37 22.17,57.62 28.92,49.87 27.92,42.37 19.42,43.62 29.17,37.62 30.42,37.62 36.92,33.87 26.82,31.87 28.17,37.12 33.42,36.12 34.17,32.87 25.17,34.12 24.42,34.12 23.92,33.87 23.92,33.12 23.92,32.37 24.42,31.87 25.17,31.87 25.92,31.87 30.92,29.87 23.82,37.77 25.32,37.87 26.52,37.77 26.62,34.17 25.52,30.97 25.62,30.07 24.12,28.07 22.82,26.77 22.72,25.57 29.02,29.97 28.92,27.97 28.72,26.77 27.82,25.67 29.82,24.07 31.07,24.72 27.32,23.87 26.82,24.77 25.92,23.77 22.72,23.97 20.92,19.87 20.17,19.62 19.52,20.17 30.72,19.57 33.52,19.47 33.62,23.37 32.82,22.67 33.72,21.97 22.22,16.97 22.22,14.67 39.82,15.07 40.67,13.87 40.82,19.67 44.92,14.62 51.42,34.37 19.32,3.87 17.67,28.12 21.72,19.77 21.72,19.17
  pour Top (rank 2): 25.82,84.22 31.07,84.22 31.57,84.67 36.72,84.67 41.82,84.57 42.12,84.67 42.32,84.97 42.42,85.17 42.42,85.57 42.72,85.97 45.32,85.87 45.42,85.67 45.42,84.97 45.62,84.57 45.82,84.47 46.12,84.37 47.12,84.37 50.02,84.17 51.72,83.97 53.32,83.67 54.82,83.27 55.72,82.87 56.22,82.47 56.52,82.07 56.72,81.47 56.82,80.77 56.82,74.97 56.42,74.47 56.32,74.07 56.32,69.27 56.42,68.87 56.82,68.47 56.82,39.97 56.32,39.47 56.32,33.97 56.82,33.57 56.82,4.87 56.72,3.47 56.52,2.67 56.12,2.17 55.52,1.77 54.22,1.27 52.92,0.97 51.62,0.77 48.72,0.47 44.72,0.27 43.62,0.27 43.32,0.37 38.32,0.27 38.02,0.17 36.62,0.07 20.12,0.07 18.72,0.17 18.52,0.27 13.52,0.37 13.22,0.27 10.82,0.37 7.02,0.57 3.92,0.97 2.32,1.37 1.32,1.77 0.72,2.17 0.42,2.47 0.22,2.97 0.12,3.47 0.02,4.47 0.02,33.57 0.42,33.97 0.52,34.27 0.52,39.27 0.32,39.67 0.12,39.97 0.02,40.07 0.02,68.47 0.32,68.77 0.52,69.17 0.52,74.37 0.02,74.87 0.02,80.27 0.12,81.27 0.42,82.27 0.72,82.57 1.72,83.17 3.02,83.57 4.52,83.87 7.02,84.17 9.92,84.37 10.82,84.37 11.22,84.57 11.42,84.87 11.42,85.67 11.52,85.87 14.12,85.97 14.42,85.67 14.42,85.07 14.62,84.77 14.92,84.57 15.52,84.57 19.92,84.67 25.17,84.67 25.37,84.42
  pour Bottom (rank 2): 25.82,84.27 31.02,84.27 31.42,84.47 31.62,84.67 36.72,84.67 41.82,84.57 42.12,84.67 42.32,84.97 42.42,85.17 42.42,85.57 42.72,85.97 45.32,85.87 45.42,85.67 45.42,84.97 45.62,84.57 45.82,84.47 46.12,84.37 47.12,84.37 50.02,84.17 51.72,83.97 53.32,83.67 54.82,83.27 55.72,82.87 56.22,82.47 56.52,82.07 56.72,81.47 56.82,80.77 56.82,74.97 56.42,74.47 56.32,74.07 56.32,69.27 56.42,68.87 56.82,68.47 56.82,39.97 56.32,39.47 56.32,33.97 56.82,33.57 56.82,4.87 56.72,3.47 56.52,2.67 56.12,2.17 55.52,1.77 54.22,1.27 52.92,0.97 51.62,0.77 48.72,0.47 44.72,0.27 43.62,0.27 43.32,0.37 38.32,0.27 38.02,0.17 36.62,0.07 20.12,0.07 18.72,0.17 18.52,0.27 13.52,0.37 13.22,0.27 10.82,0.37 7.02,0.57 3.92,0.97 2.32,1.37 1.32,1.77 0.72,2.17 0.42,2.47 0.22,2.97 0.12,3.47 0.02,4.47 0.02,33.57 0.42,33.97 0.52,34.27 0.52,39.27 0.32,39.67 0.12,39.97 0.02,40.07 0.02,68.47 0.32,68.77 0.52,69.17 0.52,74.37 0.02,74.87 0.02,80.27 0.12,81.27 0.42,82.27 0.72,82.57 1.72,83.17 3.02,83.57 4.52,83.87 7.02,84.17 9.92,84.37 10.82,84.37 11.22,84.57 11.42,84.87 11.42,85.67 11.52,85.87 14.12,85.97 14.42,85.67 14.42,85.07 14.62,84.77 14.92,84.57 15.52,84.57 19.92,84.67 25.32,84.67 25.62,84.37
HSIC_DAT  (via drill 0.25)
  Top 0.35: P100.5 v45.92,13.12
  Bottom 0.35: v45.92,13.12 P102.5
HSIC_STB  (via drill 0.25)
  Top 0.35: P100.3 v46.92,13.12
  Bottom 0.35: v46.92,13.12 P102.3
ILIM
  Top 0.1: R533.2
  Top 0.25: U520.10 27.92,22.07 28.76,22.91 R533.2
LED_A
  Top 0.1: R122.2
  Top 0.2: D123.P$1 R122.2
LED_K
  Top 0.2: D123.P$2 26.62,5.87 26.22,5.47 26.22,5.37 Q121.3
OTG
  Top 0.25: U520.8 28.92,21.67 29.32,22.07 R535.2
PA0  (via drill 0.25)
  Top 0.35: P100.12 v42.92,6.37
  Bottom 0.35: v42.92,6.37 P102.12
PA1  (via drill 0.25)
  Top 0.35: P100.14 v41.92,6.37
  Bottom 0.35: v41.92,6.37 P102.14
PA2  (via drill 0.25)
  Top 0.35: P100.8 v44.92,6.37
  Bottom 0.35: v44.92,6.37 P102.8
PA3  (via drill 0.25)
  Top 0.35: P100.10 v43.92,6.37
  Bottom 0.35: v43.92,6.37 P102.10
PA4  (via drill 0.25)
  Top 0.35: P100.28 v34.92,6.37
  Bottom 0.35: v34.92,6.37 P102.28
PA5  (via drill 0.25)
  Top 0.35: P100.26 v35.92,6.37
  Bottom 0.35: v35.92,6.37 P102.26
PA6  (via drill 0.25)
  Top 0.35: P100.22 v37.92,6.37
  Bottom 0.35: v37.92,6.37 P102.22
PA7  (via drill 0.25)
  Top 0.35: P100.20 v38.92,6.37
  Bottom 0.35: v38.92,6.37 P102.20
PA9  (via drill 0.25)
  Top 0.35: P100.32 v32.92,6.37
  Bottom 0.35: v32.92,6.37 P102.32
PA10  (via drill 0.25)
  Top 0.35: P100.16 v40.92,6.37
  Bottom 0.35: v40.92,6.37 P102.16
PA15  (via drill 0.25)
  Top 0.35: P100.30 v33.92,6.37
  Bottom 0.35: v33.92,6.37 P102.30
PB2  (via drill 0.25)
  Top 0.2: v45.92,6.37 46.62,5.67 48.32,5.67 51.07,8.42 v51.07,12.57 | v51.07,14.72 51.07,18.27 39.97,29.37 R517.2 R518.1
  Top 0.35: P100.6 v45.92,6.37
  Bottom 0.15: v51.07,14.72 v51.07,12.57
  Bottom 0.35: v45.92,6.37 P102.6
PB10  (via drill 0.25)
  Top 0.1: P100.54 21.92,6.97 v21.52,6.57 20.82,5.87 19.17,5.87 18.42,5.12 17.92,5.12 | 17.92,5.12 7.37,5.12 4.92,7.57 4.92,15.12 5.25,15.45 EE_SCL.TP 7.5,15.45 8.12,16.07 8.12,16.67 8.3,16.85 D125.P$1 U105.P$6 | v17.93,5.67 17.93,5.15 17.92,5.12 | v50.32,4.67 50.02,4.97 49.43,4.97 47.96,3.51 21.06,3.51 20.52,2.97 18.43,2.97 v17.93,3.47 | v23.17,36.37 23.42,36.12 U500.3 | U520.5 30.82,20.27 v31.02,20.07 31.32,20.37 D537.P$1
  Bottom 0.1: v23.17,36.37 20.82,36.37 20.51,36.69 20.46,36.69 20.46,38.01 23.79,41.34 32.31,41.34 34.89,38.76 34.89,25.89 30.62,21.62 30.62,20.47 v31.02,20.07 31.57,20.62 42.42,20.62 48.82,14.22 48.82,7.28 49.79,6.32 49.79,5.21 v50.32,4.67 | v17.93,5.67 v17.93,3.47
  Bottom 0.35: P102.54 21.92,6.97 v21.52,6.57
PB11  (via drill 0.25)
  Top 0.1: P100.52 22.92,7.67 22.82,7.57 22.82,6.67 v22.72,6.57 22.27,6.12 21.42,6.12 20.92,5.62 19.42,5.62 18.67,4.87 18.52,4.87 | 18.52,4.87 7.22,4.87 4.67,7.42 4.67,17.12 5.54,17.99 EE_SDA.TP 7.06,16.85 D126.P$1 8.17,17.6 U105.P$5 | v50.32,5.37 50.07,5.17 49.32,5.17 47.86,3.71 20.96,3.71 20.42,3.17 19.32,3.17 18.52,3.97 18.52,4.87 | U500.4 22.7,35.62 v22.67,35.65 | U520.6 30.84,20.77 30.93,20.86 v31.12,20.86 31.43,20.86 D536.P$1
  Bottom 0.1: v22.67,35.65 22.2,36.12 20.62,36.12 20.17,36.57 20.17,38.12 23.67,41.62 32.42,41.62 35.17,38.87 35.17,25.77 31.12,21.72 v31.12,20.86 42.61,20.86 49.12,14.35 49.12,7.41 50.02,6.51 50.02,5.67 v50.32,5.37
  Bottom 0.35: P102.52 22.92,6.77 v22.72,6.57
PC0  (via drill 0.25)
  Top 0.35: P100.4 v46.92,6.37
  Bottom 0.35: P102.4 v46.92,6.37
PC1  (via drill 0.25)
  Top 0.35: P100.2 v47.92,6.37
  Bottom 0.35: P102.2 v47.92,6.37
PC3  (via drill 0.25)
  Top 0.1: 12.92,8.87 P100.72 12.92,8.12
  Top 0.35: 12.92,8.12 v12.92,6.37
  Bottom 0.35: P102.72 v12.92,6.37
PC7  (via drill 0.25)
  Top 0.1: U520.7 29.42,21.47 29.62,21.67 32.42,21.67 | 32.42,21.67 32.79,21.67 | v33.52,21.27 33.25,21 D532.P$1 R531.2 32.42,21.67 | P100.23 36.92,9.97 37.42,9.47 48.22,9.47 50,11.25 v50,13.12
  Top 0.35: v36.92,13.12 P100.23
  Bottom 0.1: v33.52,21.27 33.62,21.17 42.72,21.17 49.42,14.47 49.42,13.7 v50,13.12
  Bottom 0.35: P102.23 v36.92,13.12
PC8  (via drill 0.25)
  Top 0.35: P100.18 v39.92,6.37
  Bottom 0.35: v39.92,6.37 P102.18
PC9  (via drill 0.25)
  Top 0.3: P100.33 v31.92,13.12
  Bottom 0.35: v31.92,13.12 P102.33
PC12  (via drill 0.25)
  Top 0.35: 11.92,8.37 P100.74 v11.92,6.37
  Bottom 0.35: P102.74 v11.92,6.37
PC14  (via drill 0.25)
  Top 0.35: P100.25 v35.92,13.12
  Bottom 0.35: v35.92,13.12 P102.25
PC15  (via drill 0.25)
  Top 0.35: P100.27 v34.92,13.12
  Bottom 0.35: v34.92,13.12 P102.27
PD6  (via drill 0.25)
  Top 0.35: P100.24 v36.92,6.37
  Bottom 0.35: v36.92,6.37 P102.24
PD7  (via drill 0.25)
  Top 0.35: P100.31 v32.92,13.12
  Bottom 0.35: v32.92,13.12 P102.31
PE7  (via drill 0.25)
  Top 0.35: P100.29 v33.92,13.12
  Bottom 0.35: v33.92,13.12 P102.29
PG9  (via drill 0.25)
  Top 0.1: v10.92,6.37 9.92,5.37 7.42,5.37 5.17,7.62 5.17,12.37 5.71,12.91 EE_WP.TP 6.71,12.91 9.65,15.85 D124.P$1 R108.2 9.55,16.44 9.32,16.67 9.32,17.37 9.17,17.52 U105.P$7
  Top 0.35: P100.76 v10.92,6.37
  Bottom 0.35: P102.76 v10.92,6.37
PG10  (via drill 0.25)
  Top 0.1: Q539.1 v32.02,24.67 | v32.02,26.17 31.92,26.27 22.72,26.27 10.87,14.42 9.02,14.42 7.92,13.32 7.92,6.37 8.42,5.87 9.42,5.87 v9.92,6.37
  Top 0.2: R540.1 32.55,23.97 Q539.1
  Top 0.35: P100.78 v9.92,6.37
  Bottom 0.15: v32.02,26.17 v32.02,24.67
  Bottom 0.35: v9.92,6.37 P102.78
PG12  (via drill 0.25)
  Top 0.1: P100.80 8.92,8.87 8.52,9.27 8.52,13.27 8.97,13.72 11.17,13.72 v11.67,14.22
  Top 0.25: U500.8 v28.17,36.12
  Top 0.35: 8.92,8.37 P100.80 v8.92,6.37
  Bottom 0.1: v28.17,36.12 24.67,36.12 12.92,24.37 12.92,15.47 v11.67,14.22
  Bottom 0.35: v8.92,6.37 P102.80
PGND  (via drill 0.25)
  Top 0.1: v27.17,20.37 U520.G1
  Bottom 0.1: E548.2 U520.G1
  other vias: 30.82,16.07 31.32,16.07 31.72,14.97 25.67,18.62 25.67,18.12 25.67,17.62 29.17,20.37 29.17,18.62 27.17,18.62 23.02,22.97
  pour Bottom: 32.37,18.07 32.37,15.27 31.62,14.52 28.67,14.52 28.57,14.62 28.57,15.42 28.37,15.62 26.27,15.62 25.97,15.32 25.97,14.57 25.72,14.32 22.77,14.32 22.67,14.42 22.67,17.12 23.27,17.12 23.57,17.42 23.57,18.32 23.07,18.82 22.72,18.82 22.37,19.17 22.37,22.72 22.67,23.12 23.32,23.12 23.62,22.82 25.82,22.82 25.92,22.92 26.57,22.92 26.57,21.07 26.72,20.92 29.57,20.92 29.57,18.52 31.92,18.52
  pour Top: 22.87,23.12 23.12,23.12 23.27,22.97 23.27,21.52 23.17,21.42 22.87,21.42 22.77,21.52 22.77,23.02
  pour Top: 24.37,18.92 26.57,18.92 26.57,18.17 25.52,17.12 24.37,17.12
  pour Top: 31.67,14.62 30.77,14.62 30.57,14.82 30.57,16.12 30.67,16.22 32.17,16.22 32.37,16.02 32.37,15.32
PH0  (via drill 0.25)
  Top 0.35: P100.70 v13.92,6.37
  Bottom 0.35: P102.70 v13.92,6.37
PM_SW
  pour Top: 27.57,17.92 26.77,17.92 25.27,16.42 24.82,16.42 24.67,16.27 24.67,14.37 25.52,14.37 25.67,14.52 25.67,15.52 26.22,16.07 26.72,16.07 26.72,16.67 26.77,16.72 27.27,16.72 27.57,17.02
PM_TS
  Top 0.25: R546.1 R547.1 27.17,22.37 27.4,22.14 27.4,21.37 U520.11
PMID
  pour Top: 28.77,17.87 29.07,17.87 29.07,17.17 29.77,16.47 29.77,14.57 29.07,14.57 29.07,15.67 28.77,15.97
POWERGOOD
  Top 0.1: Q121.1 24.31,5.67 U120.2
PSEL
  Top 0.25: U520.2 30.72,18.77 31.57,19.62 R534.2
TE  (via drill 0.25)
  Top 0.3: P100.35 v30.92,13.12
  Bottom 0.35: v30.92,13.12 P102.35
THERM_PWR
  Top 0.25: R503.1 U500.9
USB_DN  (via drill 0.25)
  Top 0.1: v10.12,9.8 10.27,9.95 10.27,10.55 9.92,10.9 P100.77 9.92,11.52
  Bottom 0.1: P102.77 9.92,10.75 10.27,10.4 10.27,9.95 v10.12,9.8
USB_DP  (via drill 0.25)
  Top 0.1: P100.75 10.92,10.9 10.57,10.55 10.57,10 v10.77,9.8
  Bottom 0.1: P102.75 10.92,10.75 10.57,10.4 10.57,10 v10.77,9.8
VBUS  (via drill 0.25)
  Top 0.3: P100.11 P102.11
  Top 0.7: P102.11 v42.92,13.62
  Bottom 0.4: P102.11 42.92,12.77
  Bottom 0.8: 42.92,12.77 v42.92,13.12 v42.92,13.62
  other vias: 32.82,17.27 33.02,17.77 33.52,17.87
  pour Bottom: 33.82,19.07 41.92,19.07 44.37,16.62 44.37,14.37 43.47,13.47 43.47,13.22 43.17,12.92 42.72,12.92 40.12,15.52 33.97,15.52 32.67,16.82 32.67,17.92
  pour Top: 33.77,18.42 33.77,16.82 30.32,16.82 29.77,17.37 29.77,18.42
VREGN
  Top 0.2: R538.1 30.42,25.37
  Top 0.25: 28.03,14.87 28.02,14.86 28.02,14.67 28.62,14.07 33.32,14.07 34.42,15.17 34.42,19.97 | 34.42,19.97 33.32,19.97 32.97,19.62 R534.1 | 34.42,19.97 34.42,23.67 32.72,25.37 30.42,25.37 28.92,25.37 27.92,24.37 R546.2
  pour Top: 28.27,17.87 28.57,17.87 28.57,14.72 28.47,14.62 27.57,14.62 27.57,15.62 28.27,16.32
VSYS  (via drill 0.25)
  Top 0.35: P100.17 v39.92,13.12
  Bottom 0.35: v39.92,13.12 P102.17
  other vias: 22.92,17.97 22.42,17.97 21.92,17.97
  pour Bottom: 39.47,10.82 39.67,10.62 40.02,10.62 40.47,11.07 40.47,13.42 40.27,13.62 40.27,13.92 39.32,14.87 33.27,14.87 32.82,14.42 32.12,14.42 31.82,14.12 27.97,14.12 27.52,13.67 27.12,13.67 26.87,13.92 22.47,13.92 21.77,14.62 21.77,17.12 22.02,17.37 22.92,17.37 23.17,17.62 23.17,18.17 22.72,18.62 21.32,18.62 20.32,17.62 20.32,14.22 21.42,13.12 26.42,13.12 26.62,12.92 27.22,12.92 27.42,13.12 29.42,13.12 29.97,13.67 39.07,13.67 39.47,13.27
  pour Top: 26.62,19.92 25.07,19.92 23.97,21.02 23.27,21.02 23.27,19.22 22.77,19.22 22.77,18.92 22.47,18.62 22.02,18.62 21.77,18.37 21.77,17.62 21.92,17.47 22.42,17.47 22.77,17.12 22.77,14.42 23.97,14.42 23.97,18.92 24.22,19.17 26.62,19.17
(copper drawn outside any net)
  shapes: Bottom circle x12, Top circle x12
